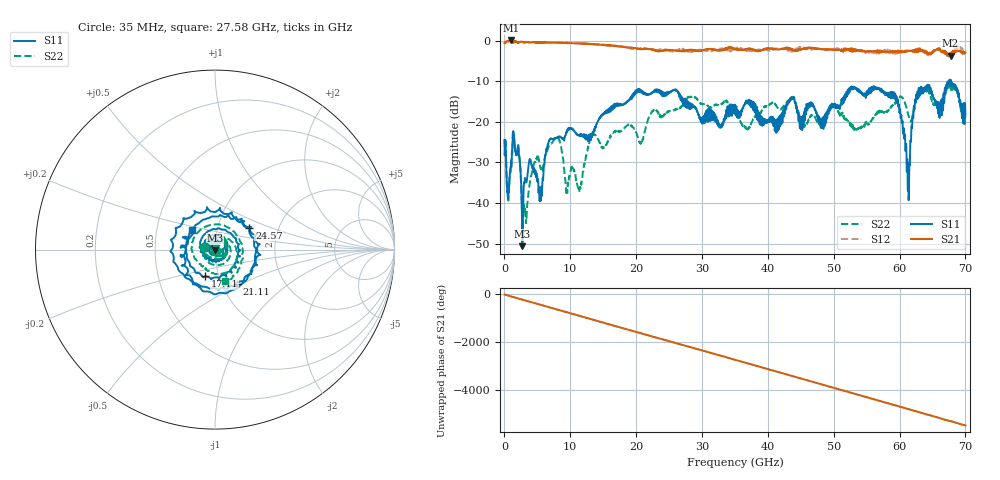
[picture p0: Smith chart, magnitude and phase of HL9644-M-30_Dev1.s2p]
! 7/2/2021 9:52:14 AM
! H:\PRODUCTION_DATA\TEMP_S2P.S2P
! CHANNEL.1
! TR.MEASUREMENT
! CORRECTED.DATA
# GHZ S RI R 50.0
! FREQ.GHZ  S11RE  S11IM  S21RE  S21IM  S12RE  S12IM  S22RE  S22IM
!; PortSelection: Port_12
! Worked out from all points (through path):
!   2000 points, 35 MHz to 70 GHz, reference 50 ohm
!   highest |S21| = 0.03 dB at 1.015 GHz (marker M1); lowest = -3.7 dB at 67.76 GHz (marker M2)
!   group delay of S21, straight-line fit = 217 ps
!   lowest |S11| = -50.6 dB at 2.73 GHz (marker M3), VSWR 1.01, Z = 50 - j0.29 ohm
!   |S11| at or under -10 dB: start of sweep to 67.43 GHz; 67.46771 GHz to 67.5854 GHz (117.7 MHz wide, 0.174 % of centre); 67.81 GHz to end of sweep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
!   |S22| runs from -47.3 to -11.2 dB; largest |S21 - S12| = 0.11
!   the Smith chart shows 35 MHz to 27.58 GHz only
!   S11 on the Smith chart (normalised r, x): 35 MHz: 0.89, +0.03; 17.11 GHz: 0.86, -0.26; 21.11 GHz: 1.17, -0.47; 24.57 GHz: 1.42, +0.37; 27.58 GHz: 0.75, +0.17
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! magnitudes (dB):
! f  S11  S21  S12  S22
! 35 MHz  -24.5  -0.6  -0.6  -24.4
! 1.015 GHz  -29.7  0.0  -0.1  -29.6
! 2.065 GHz  -26.1  -0.5  -0.6  -26.3
! 2.73 GHz  -50.6  -0.3  -0.3  -45.4
! 3.99 GHz  -29.4  -0.5  -0.5  -33.8
! 5.53 GHz  -38.7  -0.5  -0.5  -31.3
! 7.84 GHz  -24.0  -0.5  -0.5  -24.0
! 9.45 GHz  -22.7  -0.5  -0.6  -36.6
! 11.72 GHz  -23.1  -0.7  -0.7  -34.8
! 13.3 GHz  -23.8  -0.9  -0.9  -23.5
! 17.11 GHz  -16.1  -1.4  -1.3  -22.3
! 21.11 GHz  -12.9  -2.1  -1.8  -23.8
! 23.38 GHz  -12.6  -2.5  -2.5  -17.6
! 24.57 GHz  -12.9  -2.4  -2.3  -17.8
! 27.58 GHz  -15.4  -2.5  -2.5  -14.7
! 35.03 GHz  -15.8  -2.0  -2.1  -16.1
! 46.69 GHz  -15.5  -1.8  -2.1  -18.3
! 58.34 GHz  -13.9  -2.9  -2.5  -17.2
! 61.25 GHz  -36.8  -2.5  -2.5  -17.7
! 62.79 GHz  -13.3  -2.3  -2.2  -12.9
! 67.76 GHz  -10.0  -3.7  -3.0  -11.3
! 70 GHz  -18.7  -3.0  -2.7  -17.9
